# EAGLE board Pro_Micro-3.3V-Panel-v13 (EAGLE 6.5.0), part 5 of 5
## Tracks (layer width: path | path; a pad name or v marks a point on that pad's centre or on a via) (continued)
VCC  (via drill 0.25) (continued)
  Top 0.203: SJ1.2 7.72,37.75 8.13,37.34 8.76,37.34 9.21,36.89 11.37,36.89 12.06,36.2 12.06,35.52 R2.2 12.78,34.78 R11.2 11.93,32.51 C13.A | C3.2 20.51,15.84 20.85,15.49 20.85,13.22 D3.A | 11.14,13.88 C10.1 | 11.38,12.48 D1.A 11.32,12.55 C10.1 | 11.99,19.17 11.59,18.76 11.33,18.76 10.55,17.98 v10.55,16.75 10.41,16.61 10.41,14.78 C10.1 | 19.82,15.84 C3.2 | 17.06,16.73 17.39,16.4 17.39,14.94 arc90 17.44,14.88 | U3.34 20.33,21.92 21.33,21.92 v21.34,21.94 | C13.A 12.31,30.11 | 15.95,27.65 15.95,29.96 15.59,30.32 13.61,30.32 13.4,30.11 C13.A | 15.95,27.65 arc90 15.84,27.76 U2.5 | 17.14,27.19 18.2,27.19 18.41,26.98 18.41,26.5 18.69,26.22 20.82,26.22 v21.51,26.92 23.04,28.45 JP6.4 23.23,28.45 | 17.14,27.19 16.18,27.19 15.95,27.42 15.95,27.65 | 17.14,27.19 17.07,27.12 17.07,25.64 16.71,25.28 | v16.55,14.88 17.44,14.88 | 17.44,14.88 19.11,14.88 C3.2
  Bottom 0.203: v10.55,16.75 10.41,16.61 10.41,15.49 10.97,14.93 10.97,13.48 11.4,13.05 14.43,13.05 16.27,14.88 v16.55,14.88 arc90 v16.56,14.89 16.56,19.27 14.83,21 14.83,21.41 15.56,22.14 15.94,22.14 16.94,23.14 17.12,23.14 17.59,22.67 | v21.34,21.94 20.61,21.94 20.52,22.03 18.23,22.03 17.59,22.67 | v21.51,26.92 21.51,26.59 17.59,22.67
VCC1  (via drill 0.25)
  Top 0.203: SJ2.2 26,37.75 26.42,37.34 27.05,37.34 27.5,36.89 29.65,36.89 30.35,36.2 30.35,35.52 R3.2 31.06,34.78 R1.2 30.21,32.51 C8.A | C9.2 38.8,15.84 39.14,15.49 39.14,13.22 D4.A | 29.43,13.88 C7.1 | 29.67,12.48 D5.A 29.6,12.55 C7.1 | 30.28,19.17 29.88,18.76 29.62,18.76 28.84,17.98 v28.84,16.75 28.7,16.61 28.7,14.78 C7.1 | 38.11,15.84 C9.2 | 35.35,16.73 35.67,16.4 35.67,14.94 arc90 35.73,14.88 | U4.34 38.61,21.92 39.61,21.92 v39.63,21.94 | C8.A 30.6,30.11 | 34.23,27.65 34.23,29.96 33.87,30.32 31.9,30.32 31.68,30.11 C8.A | 34.23,27.65 arc90 34.12,27.76 U1.5 | 35.42,27.19 36.49,27.19 36.7,26.98 36.7,26.5 36.98,26.22 39.11,26.22 v39.8,26.92 41.33,28.45 JP3.4 41.52,28.45 | 35.42,27.19 34.47,27.19 34.23,27.42 34.23,27.65 | 35.42,27.19 35.36,27.12 35.36,25.64 35,25.28 | v34.84,14.88 35.73,14.88 | 35.73,14.88 37.4,14.88 C9.2
  Bottom 0.203: v28.84,16.75 28.7,16.61 28.7,15.49 29.26,14.93 29.26,13.48 29.69,13.05 32.72,13.05 34.55,14.88 v34.84,14.88 arc90 34.84,14.89 34.84,19.27 33.12,21 33.12,21.41 33.85,22.14 34.23,22.14 35.23,23.14 35.41,23.14 35.88,22.67 | v39.63,21.94 38.9,21.94 38.81,22.03 36.52,22.03 35.88,22.67 | v39.8,26.92 39.8,26.59 35.88,22.67
VCC2  (via drill 0.25)
  Top 0.203: SJ3.2 44.29,37.75 44.7,37.34 45.34,37.34 45.78,36.89 47.94,36.89 48.64,36.2 48.64,35.52 R14.2 49.35,34.78 R13.2 48.5,32.51 C20.A | C21.2 57.09,15.84 57.43,15.49 57.43,13.22 D7.A | 47.71,13.88 C18.1 | 47.95,12.48 D8.A 47.89,12.55 C18.1 | 48.57,19.17 48.16,18.76 47.91,18.76 47.13,17.98 v47.13,16.75 46.99,16.61 46.99,14.78 C18.1 | 56.4,15.84 C21.2 | 53.64,16.73 53.96,16.4 53.96,14.94 arc90 54.02,14.88 | U6.34 56.9,21.92 57.9,21.92 v57.92,21.94 | C20.A 48.88,30.11 | 52.52,27.65 52.52,29.96 52.16,30.32 50.19,30.32 49.97,30.11 C20.A | 52.52,27.65 arc90 52.41,27.76 U5.5 | 53.71,27.19 54.78,27.19 54.99,26.98 54.99,26.5 55.26,26.22 57.39,26.22 v58.09,26.92 59.62,28.45 JP9.4 59.81,28.45 | 53.71,27.19 52.75,27.19 52.52,27.42 52.52,27.65 | 53.71,27.19 53.65,27.12 53.65,25.64 53.29,25.28 | v53.12,14.88 54.02,14.88 | 54.02,14.88 55.69,14.88 C21.2
  Bottom 0.203: v47.13,16.75 46.99,16.61 46.99,15.49 47.55,14.93 47.55,13.48 47.98,13.05 51.01,13.05 52.84,14.88 v53.12,14.88 arc90 53.13,14.89 53.13,19.27 51.41,21 51.41,21.41 52.14,22.14 52.52,22.14 53.52,23.14 53.69,23.14 54.17,22.67 | v57.92,21.94 57.19,21.94 57.1,22.03 54.81,22.03 54.17,22.67 | v58.09,26.92 58.09,26.59 54.17,22.67
VCC3  (via drill 0.25)
  Top 0.203: SJ4.2 62.58,37.75 62.99,37.34 63.63,37.34 64.07,36.89 66.23,36.89 66.93,36.2 66.93,35.52 R20.2 67.64,34.78 R19.2 66.79,32.51 C29.A | C30.2 75.38,15.84 75.72,15.49 75.72,13.22 D10.A | 66,13.88 C28.1 | 66.24,12.48 D11.A 66.18,12.55 C28.1 | 66.86,19.17 66.45,18.76 66.2,18.76 65.42,17.98 v65.42,16.75 65.28,16.61 65.28,14.78 C28.1 | 74.69,15.84 C30.2 | 71.92,16.73 72.25,16.4 72.25,14.94 arc90 72.31,14.88 | U8.34 75.19,21.92 76.19,21.92 v76.21,21.94 | C29.A 67.17,30.11 | 70.81,27.65 70.81,29.96 70.45,30.32 68.47,30.32 68.26,30.11 C29.A | 70.81,27.65 arc90 70.7,27.76 U7.5 | 72,27.19 73.07,27.19 73.27,26.98 73.27,26.5 73.55,26.22 75.68,26.22 v76.38,26.92 77.91,28.45 JP13.4 78.09,28.45 | 72,27.19 71.04,27.19 70.81,27.42 70.81,27.65 | 72,27.19 71.94,27.12 71.94,25.64 71.58,25.28 | v71.41,14.88 72.31,14.88 | 72.31,14.88 73.97,14.88 C30.2
  Bottom 0.203: v65.42,16.75 65.28,16.61 65.28,15.49 65.84,14.93 65.84,13.48 66.27,13.05 69.3,13.05 71.13,14.88 v71.41,14.88 arc90 v71.42,14.89 71.42,19.27 69.69,21 69.69,21.41 70.43,22.14 70.81,22.14 71.8,23.14 71.98,23.14 72.45,22.67 | v76.21,21.94 75.48,21.94 75.39,22.03 73.1,22.03 72.45,22.67 | v76.38,26.92 76.38,26.59 72.45,22.67
VCC4  (via drill 0.25)
  Top 0.203: SJ5.2 80.87,37.75 81.28,37.34 81.92,37.34 82.36,36.89 84.52,36.89 85.22,36.2 85.22,35.52 R26.2 85.93,34.78 R25.2 85.08,32.51 C38.A | C39.2 93.66,15.84 94,15.49 94,13.22 D13.A | 84.29,13.88 C37.1 | 84.53,12.48 D14.A 84.47,12.55 C37.1 | 85.15,19.17 84.74,18.76 84.48,18.76 83.71,17.98 v83.71,16.75 83.57,16.61 83.57,14.78 C37.1 | 92.98,15.84 C39.2 | 90.21,16.73 90.54,16.4 90.54,14.94 arc90 90.59,14.88 | U10.34 93.48,21.92 94.48,21.92 v94.5,21.94 | C38.A 85.46,30.11 | 89.1,27.65 89.1,29.96 88.74,30.32 86.76,30.32 86.55,30.11 C38.A | 89.1,27.65 arc90 88.99,27.76 U9.5 | 90.29,27.19 91.36,27.19 91.56,26.98 91.56,26.5 91.84,26.22 93.97,26.22 v94.66,26.92 96.19,28.45 JP17.4 96.38,28.45 | 90.29,27.19 89.33,27.19 89.1,27.42 89.1,27.65 | 90.29,27.19 90.23,27.12 90.23,25.64 89.86,25.28 | v89.7,14.88 90.59,14.88 | 90.59,14.88 92.26,14.88 C39.2
  Bottom 0.203: v83.71,16.75 83.57,16.61 83.57,15.49 84.12,14.93 84.12,13.48 84.55,13.05 87.58,13.05 89.42,14.88 v89.7,14.88 arc90 v89.71,14.89 89.71,19.27 87.98,21 87.98,21.41 88.72,22.14 89.09,22.14 90.09,23.14 90.27,23.14 90.74,22.67 | v94.5,21.94 93.76,21.94 93.67,22.03 91.38,22.03 90.74,22.67 | v94.66,26.92 94.66,26.59 90.74,22.67
VCC5  (via drill 0.25)
  Top 0.203: SJ6.2 99.16,37.75 99.57,37.34 100.2,37.34 100.65,36.89 102.81,36.89 103.5,36.2 103.5,35.52 R32.2 104.22,34.78 R31.2 103.36,32.51 C47.A | C48.2 111.95,15.84 112.29,15.49 112.29,13.22 D16.A | 102.58,13.88 C46.1 | 102.82,12.48 D17.A 102.76,12.55 C46.1 | 103.43,19.17 103.03,18.76 102.77,18.76 101.99,17.98 v101.99,16.75 101.85,16.61 101.85,14.78 C46.1 | 111.26,15.84 C48.2 | 108.5,16.73 108.83,16.4 108.83,14.94 arc90 108.88,14.88 | U12.34 111.77,21.92 112.77,21.92 v112.78,21.94 | C47.A 103.75,30.11 | 107.39,27.65 107.39,29.96 107.03,30.32 105.05,30.32 104.84,30.11 C47.A | 107.39,27.65 arc90 107.28,27.76 U11.5 | 108.58,27.19 109.64,27.19 109.85,26.98 109.85,26.5 110.13,26.22 112.26,26.22 v112.95,26.92 114.48,28.45 JP21.4 114.67,28.45 | 108.58,27.19 107.62,27.19 107.39,27.42 107.39,27.65 | 108.58,27.19 108.51,27.12 108.51,25.64 108.15,25.28 | v107.99,14.88 108.88,14.88 | 108.88,14.88 110.55,14.88 C48.2
  Bottom 0.203: v101.99,16.75 101.85,16.61 101.85,15.49 102.41,14.93 102.41,13.48 102.84,13.05 105.87,13.05 107.7,14.88 v107.99,14.88 arc90 v108,14.89 108,19.27 106.27,21 106.27,21.41 107,22.14 107.38,22.14 108.38,23.14 108.56,23.14 109.03,22.67 | v112.78,21.94 112.05,21.94 111.96,22.03 109.67,22.03 109.03,22.67 | v112.95,26.92 112.95,26.59 109.03,22.67
VCC6  (via drill 0.25)
  Top 0.203: SJ7.2 7.72,74.58 8.13,74.17 8.76,74.17 9.21,73.72 11.37,73.72 12.06,73.03 12.06,72.35 R38.2 12.78,71.61 R37.2 11.93,69.34 C56.A | C57.2 20.51,52.67 20.85,52.32 20.85,50.05 D19.A | 11.14,50.71 C55.1 | 11.38,49.31 D20.A 11.32,49.38 C55.1 | 11.99,56 11.59,55.59 11.33,55.59 10.55,54.81 v10.55,53.58 10.41,53.44 10.41,51.61 C55.1 | 19.82,52.67 C57.2 | 17.06,53.56 17.39,53.23 17.39,51.77 arc90 17.44,51.71 | U14.34 20.33,58.75 21.33,58.75 v21.34,58.77 | C56.A 12.31,66.94 | 15.95,64.48 15.95,66.79 15.59,67.15 13.61,67.15 13.4,66.94 C56.A | 15.95,64.48 arc90 15.84,64.59 U13.5 | 17.14,64.02 18.2,64.02 18.41,63.81 18.41,63.33 18.69,63.05 20.82,63.05 v21.51,63.75 23.04,65.28 JP25.4 23.23,65.28 | 17.14,64.02 16.18,64.02 15.95,64.25 15.95,64.48 | 17.14,64.02 17.07,63.95 17.07,62.47 16.71,62.11 | v16.55,51.71 17.44,51.71 | 17.44,51.71 19.11,51.71 C57.2
  Bottom 0.203: v10.55,53.58 10.41,53.44 10.41,52.32 10.97,51.76 10.97,50.31 11.4,49.88 14.43,49.88 16.27,51.71 v16.55,51.71 arc90 v16.56,51.72 16.56,56.1 14.83,57.83 14.83,58.24 15.56,58.97 15.94,58.97 16.94,59.97 17.12,59.97 17.59,59.5 | v21.34,58.77 20.61,58.77 20.52,58.86 18.23,58.86 17.59,59.5 | v21.51,63.75 21.51,63.42 17.59,59.5
VCC7  (via drill 0.25)
  Top 0.203: SJ8.2 26,74.58 26.42,74.17 27.05,74.17 27.5,73.72 29.65,73.72 30.35,73.03 30.35,72.35 R44.2 31.06,71.61 R43.2 30.21,69.34 C65.A | C66.2 38.8,52.67 39.14,52.32 39.14,50.05 D22.A | 29.43,50.71 C64.1 | 29.67,49.31 D23.A 29.6,49.38 C64.1 | 30.28,56 29.88,55.59 29.62,55.59 28.84,54.81 v28.84,53.58 28.7,53.44 28.7,51.61 C64.1 | 38.11,52.67 C66.2 | 35.35,53.56 35.67,53.23 35.67,51.77 arc90 35.73,51.71 | U16.34 38.61,58.75 39.61,58.75 v39.63,58.77 | C65.A 30.6,66.94 | 34.23,64.48 34.23,66.79 33.87,67.15 31.9,67.15 31.68,66.94 C65.A | 34.23,64.48 arc90 34.12,64.59 U15.5 | 35.42,64.02 36.49,64.02 36.7,63.81 36.7,63.33 36.98,63.05 39.11,63.05 v39.8,63.75 41.33,65.28 JP29.4 41.52,65.28 | 35.42,64.02 34.47,64.02 34.23,64.25 34.23,64.48 | 35.42,64.02 35.36,63.95 35.36,62.47 35,62.11 | v34.84,51.71 35.73,51.71 | 35.73,51.71 37.4,51.71 C66.2
  Bottom 0.203: v28.84,53.58 28.7,53.44 28.7,52.32 29.26,51.76 29.26,50.31 29.69,49.88 32.72,49.88 34.55,51.71 v34.84,51.71 arc90 34.84,51.72 34.84,56.1 33.12,57.83 33.12,58.24 33.85,58.97 34.23,58.97 35.23,59.97 35.41,59.97 35.88,59.5 | v39.63,58.77 38.9,58.77 38.81,58.86 36.52,58.86 35.88,59.5 | v39.8,63.75 39.8,63.42 35.88,59.5
VCC8  (via drill 0.25)
  Top 0.203: SJ9.2 44.29,74.58 44.7,74.17 45.34,74.17 45.78,73.72 47.94,73.72 48.64,73.03 48.64,72.35 R50.2 49.35,71.61 R49.2 48.5,69.34 C74.A | C75.2 57.09,52.67 57.43,52.32 57.43,50.05 D25.A | 47.71,50.71 C73.1 | 47.95,49.31 D26.A 47.89,49.38 C73.1 | 48.57,56 48.16,55.59 47.91,55.59 47.13,54.81 v47.13,53.58 46.99,53.44 46.99,51.61 C73.1 | 56.4,52.67 C75.2 | 53.64,53.56 53.96,53.23 53.96,51.77 arc90 54.02,51.71 | U18.34 56.9,58.75 57.9,58.75 v57.92,58.77 | C74.A 48.88,66.94 | 52.52,64.48 52.52,66.79 52.16,67.15 50.19,67.15 49.97,66.94 C74.A | 52.52,64.48 arc90 52.41,64.59 U17.5 | 53.71,64.02 54.78,64.02 54.99,63.81 54.99,63.33 55.26,63.05 57.39,63.05 v58.09,63.75 59.62,65.28 JP33.4 59.81,65.28 | 53.71,64.02 52.75,64.02 52.52,64.25 52.52,64.48 | 53.71,64.02 53.65,63.95 53.65,62.47 53.29,62.11 | v53.12,51.71 54.02,51.71 | 54.02,51.71 55.69,51.71 C75.2
  Bottom 0.203: v47.13,53.58 46.99,53.44 46.99,52.32 47.55,51.76 47.55,50.31 47.98,49.88 51.01,49.88 52.84,51.71 v53.12,51.71 arc90 53.13,51.72 53.13,56.1 51.41,57.83 51.41,58.24 52.14,58.97 52.52,58.97 53.52,59.97 53.69,59.97 54.17,59.5 | v57.92,58.77 57.19,58.77 57.1,58.86 54.81,58.86 54.17,59.5 | v58.09,63.75 58.09,63.42 54.17,59.5
VCC9  (via drill 0.25)
  Top 0.203: SJ10.2 62.58,74.58 62.99,74.17 63.63,74.17 64.07,73.72 66.23,73.72 66.93,73.03 66.93,72.35 R56.2 67.64,71.61 R55.2 66.79,69.34 C83.A | C84.2 75.38,52.67 75.72,52.32 75.72,50.05 D28.A | 66,50.71 C82.1 | 66.24,49.31 D29.A 66.18,49.38 C82.1 | 66.86,56 66.45,55.59 66.2,55.59 65.42,54.81 v65.42,53.58 65.28,53.44 65.28,51.61 C82.1 | 74.69,52.67 C84.2 | 71.92,53.56 72.25,53.23 72.25,51.77 arc90 72.31,51.71 | U20.34 75.19,58.75 76.19,58.75 v76.21,58.77 | C83.A 67.17,66.94 | 70.81,64.48 70.81,66.79 70.45,67.15 68.47,67.15 68.26,66.94 C83.A | 70.81,64.48 arc90 70.7,64.59 U19.5 | 72,64.02 73.07,64.02 73.27,63.81 73.27,63.33 73.55,63.05 75.68,63.05 v76.38,63.75 77.91,65.28 JP37.4 78.09,65.28 | 72,64.02 71.04,64.02 70.81,64.25 70.81,64.48 | 72,64.02 71.94,63.95 71.94,62.47 71.58,62.11 | v71.41,51.71 72.31,51.71 | 72.31,51.71 73.97,51.71 C84.2
  Bottom 0.203: v65.42,53.58 65.28,53.44 65.28,52.32 65.84,51.76 65.84,50.31 66.27,49.88 69.3,49.88 71.13,51.71 v71.41,51.71 arc90 v71.42,51.72 71.42,56.1 69.69,57.83 69.69,58.24 70.43,58.97 70.81,58.97 71.8,59.97 71.98,59.97 72.45,59.5 | v76.21,58.77 75.48,58.77 75.39,58.86 73.1,58.86 72.45,59.5 | v76.38,63.75 76.38,63.42 72.45,59.5
VCC10  (via drill 0.25)
  Top 0.203: SJ11.2 80.87,74.58 81.28,74.17 81.92,74.17 82.36,73.72 84.52,73.72 85.22,73.03 85.22,72.35 R62.2 85.93,71.61 R61.2 85.08,69.34 C92.A | C93.2 93.66,52.67 94,52.32 94,50.05 D31.A | 84.29,50.71 C91.1 | 84.53,49.31 D32.A 84.47,49.38 C91.1 | 85.15,56 84.74,55.59 84.48,55.59 83.71,54.81 v83.71,53.58 83.57,53.44 83.57,51.61 C91.1 | 92.98,52.67 C93.2 | 90.21,53.56 90.54,53.23 90.54,51.77 arc90 90.59,51.71 | U22.34 93.48,58.75 94.48,58.75 v94.5,58.77 | C92.A 85.46,66.94 | 89.1,64.48 89.1,66.79 88.74,67.15 86.76,67.15 86.55,66.94 C92.A | 89.1,64.48 arc90 88.99,64.59 U21.5 | 90.29,64.02 91.36,64.02 91.56,63.81 91.56,63.33 91.84,63.05 93.97,63.05 v94.66,63.75 96.19,65.28 JP41.4 96.38,65.28 | 90.29,64.02 89.33,64.02 89.1,64.25 89.1,64.48 | 90.29,64.02 90.23,63.95 90.23,62.47 89.86,62.11 | v89.7,51.71 90.59,51.71 | 90.59,51.71 92.26,51.71 C93.2
  Bottom 0.203: v83.71,53.58 83.57,53.44 83.57,52.32 84.12,51.76 84.12,50.31 84.55,49.88 87.58,49.88 89.42,51.71 v89.7,51.71 arc90 v89.71,51.72 89.71,56.1 87.98,57.83 87.98,58.24 88.72,58.97 89.09,58.97 90.09,59.97 90.27,59.97 90.74,59.5 | v94.5,58.77 93.76,58.77 93.67,58.86 91.38,58.86 90.74,59.5 | v94.66,63.75 94.66,63.42 90.74,59.5
VCC11  (via drill 0.25)
  Top 0.203: SJ12.2 99.16,74.58 99.57,74.17 100.2,74.17 100.65,73.72 102.81,73.72 103.5,73.03 103.5,72.35 R68.2 104.22,71.61 R67.2 103.36,69.34 C101.A | C102.2 111.95,52.67 112.29,52.32 112.29,50.05 D34.A | 102.58,50.71 C100.1 | 102.82,49.31 D35.A 102.76,49.38 C100.1 | 103.43,56 103.03,55.59 102.77,55.59 101.99,54.81 v101.99,53.58 101.85,53.44 101.85,51.61 C100.1 | 111.26,52.67 C102.2 | 108.5,53.56 108.83,53.23 108.83,51.77 arc90 108.88,51.71 | U24.34 111.77,58.75 112.77,58.75 v112.78,58.77 | C101.A 103.75,66.94 | 107.39,64.48 107.39,66.79 107.03,67.15 105.05,67.15 104.84,66.94 C101.A | 107.39,64.48 arc90 107.28,64.59 U23.5 | 108.58,64.02 109.64,64.02 109.85,63.81 109.85,63.33 110.13,63.05 112.26,63.05 v112.95,63.75 114.48,65.28 JP45.4 114.67,65.28 | 108.58,64.02 107.62,64.02 107.39,64.25 107.39,64.48 | 108.58,64.02 108.51,63.95 108.51,62.47 108.15,62.11 | v107.99,51.71 108.88,51.71 | 108.88,51.71 110.55,51.71 C102.2
  Bottom 0.203: v101.99,53.58 101.85,53.44 101.85,52.32 102.41,51.76 102.41,50.31 102.84,49.88 105.87,49.88 107.7,51.71 v107.99,51.71 arc90 v108,51.72 108,56.1 106.27,57.83 106.27,58.24 107,58.97 107.38,58.97 108.38,59.97 108.56,59.97 109.03,59.5 | v112.78,58.77 112.05,58.77 111.96,58.86 109.67,58.86 109.03,59.5 | v112.95,63.75 112.95,63.42 109.03,59.5
VCC12  (via drill 0.25)
  Top 0.203: SJ13.2 7.72,111.41 8.13,111 8.76,111 9.21,110.55 11.37,110.55 12.06,109.86 12.06,109.18 R74.2 12.78,108.44 R73.2 11.93,106.17 C110.A | C111.2 20.51,89.5 20.85,89.15 20.85,86.88 D37.A | 11.14,87.54 C109.1 | 11.38,86.14 D38.A 11.32,86.21 C109.1 | 11.99,92.83 11.59,92.42 11.33,92.42 10.55,91.64 v10.55,90.41 10.41,90.27 10.41,88.44 C109.1 | 19.82,89.5 C111.2 | 17.06,90.39 17.39,90.06 17.39,88.6 arc90 17.44,88.54 | U26.34 20.33,95.58 21.33,95.58 v21.34,95.6 | C110.A 12.31,103.77 | 15.95,101.31 15.95,103.62 15.59,103.98 13.61,103.98 13.4,103.77 C110.A | 15.95,101.31 arc90 15.84,101.42 U25.5 | 17.14,100.85 18.2,100.85 18.41,100.64 18.41,100.16 18.69,99.88 20.82,99.88 v21.51,100.58 23.04,102.11 JP49.4 23.23,102.11 | 17.14,100.85 16.18,100.85 15.95,101.08 15.95,101.31 | 17.14,100.85 17.07,100.78 17.07,99.3 16.71,98.94 | v16.55,88.54 17.44,88.54 | 17.44,88.54 19.11,88.54 C111.2
  Bottom 0.203: v10.55,90.41 10.41,90.27 10.41,89.15 10.97,88.59 10.97,87.14 11.4,86.71 14.43,86.71 16.27,88.54 v16.55,88.54 arc90 v16.56,88.55 16.56,92.93 14.83,94.66 14.83,95.07 15.56,95.8 15.94,95.8 16.94,96.8 17.12,96.8 17.59,96.33 | v21.34,95.6 20.61,95.6 20.52,95.69 18.23,95.69 17.59,96.33 | v21.51,100.58 21.51,100.25 17.59,96.33
VCC13  (via drill 0.25)
  Top 0.203: SJ14.2 26,111.41 26.42,111 27.05,111 27.5,110.55 29.65,110.55 30.35,109.86 30.35,109.18 R80.2 31.06,108.44 R79.2 30.21,106.17 C119.A | C120.2 38.8,89.5 39.14,89.15 39.14,86.88 D40.A | 29.43,87.54 C118.1 | 29.67,86.14 D41.A 29.6,86.21 C118.1 | 30.28,92.83 29.88,92.42 29.62,92.42 28.84,91.64 v28.84,90.41 28.7,90.27 28.7,88.44 C118.1 | 38.11,89.5 C120.2 | 35.35,90.39 35.67,90.06 35.67,88.6 arc90 35.73,88.54 | U28.34 38.61,95.58 39.61,95.58 v39.63,95.6 | C119.A 30.6,103.77 | 34.23,101.31 34.23,103.62 33.87,103.98 31.9,103.98 31.68,103.77 C119.A | 34.23,101.31 arc90 34.12,101.42 U27.5 | 35.42,100.85 36.49,100.85 36.7,100.64 36.7,100.16 36.98,99.88 39.11,99.88 v39.8,100.58 41.33,102.11 JP53.4 41.52,102.11 | 35.42,100.85 34.47,100.85 34.23,101.08 34.23,101.31 | 35.42,100.85 35.36,100.78 35.36,99.3 35,98.94 | v34.84,88.54 35.73,88.54 | 35.73,88.54 37.4,88.54 C120.2
  Bottom 0.203: v28.84,90.41 28.7,90.27 28.7,89.15 29.26,88.59 29.26,87.14 29.69,86.71 32.72,86.71 34.55,88.54 v34.84,88.54 arc90 34.84,88.55 34.84,92.93 33.12,94.66 33.12,95.07 33.85,95.8 34.23,95.8 35.23,96.8 35.41,96.8 35.88,96.33 | v39.63,95.6 38.9,95.6 38.81,95.69 36.52,95.69 35.88,96.33 | v39.8,100.58 39.8,100.25 35.88,96.33
VCC14  (via drill 0.25)
  Top 0.203: SJ15.2 44.29,111.41 44.7,111 45.34,111 45.78,110.55 47.94,110.55 48.64,109.86 48.64,109.18 R86.2 49.35,108.44 R85.2 48.5,106.17 C128.A | C129.2 57.09,89.5 57.43,89.15 57.43,86.88 D43.A | 47.71,87.54 C127.1 | 47.95,86.14 D44.A 47.89,86.21 C127.1 | 48.57,92.83 48.16,92.42 47.91,92.42 47.13,91.64 v47.13,90.41 46.99,90.27 46.99,88.44 C127.1 | 56.4,89.5 C129.2 | 53.64,90.39 53.96,90.06 53.96,88.6 arc90 54.02,88.54 | U30.34 56.9,95.58 57.9,95.58 v57.92,95.6 | C128.A 48.88,103.77 | 52.52,101.31 52.52,103.62 52.16,103.98 50.19,103.98 49.97,103.77 C128.A | 52.52,101.31 arc90 52.41,101.42 U29.5 | 53.71,100.85 54.78,100.85 54.99,100.64 54.99,100.16 55.26,99.88 57.39,99.88 v58.09,100.58 59.62,102.11 JP57.4 59.81,102.11 | 53.71,100.85 52.75,100.85 52.52,101.08 52.52,101.31 | 53.71,100.85 53.65,100.78 53.65,99.3 53.29,98.94 | v53.12,88.54 54.02,88.54 | 54.02,88.54 55.69,88.54 C129.2
  Bottom 0.203: v47.13,90.41 46.99,90.27 46.99,89.15 47.55,88.59 47.55,87.14 47.98,86.71 51.01,86.71 52.84,88.54 v53.12,88.54 arc90 53.13,88.55 53.13,92.93 51.41,94.66 51.41,95.07 52.14,95.8 52.52,95.8 53.52,96.8 53.69,96.8 54.17,96.33 | v57.92,95.6 57.19,95.6 57.1,95.69 54.81,95.69 54.17,96.33 | v58.09,100.58 58.09,100.25 54.17,96.33
VCC15  (via drill 0.25)
  Top 0.203: SJ16.2 62.58,111.41 62.99,111 63.63,111 64.07,110.55 66.23,110.55 66.93,109.86 66.93,109.18 R92.2 67.64,108.44 R91.2 66.79,106.17 C137.A | C138.2 75.38,89.5 75.72,89.15 75.72,86.88 D46.A | 66,87.54 C136.1 | 66.24,86.14 D47.A 66.18,86.21 C136.1 | 66.86,92.83 66.45,92.42 66.2,92.42 65.42,91.64 v65.42,90.41 65.28,90.27 65.28,88.44 C136.1 | 74.69,89.5 C138.2 | 71.92,90.39 72.25,90.06 72.25,88.6 arc90 72.31,88.54 | U32.34 75.19,95.58 76.19,95.58 v76.21,95.6 | C137.A 67.17,103.77 | 70.81,101.31 70.81,103.62 70.45,103.98 68.47,103.98 68.26,103.77 C137.A | 70.81,101.31 arc90 70.7,101.42 U31.5 | 72,100.85 73.07,100.85 73.27,100.64 73.27,100.16 73.55,99.88 75.68,99.88 v76.38,100.58 77.91,102.11 JP61.4 78.09,102.11 | 72,100.85 71.04,100.85 70.81,101.08 70.81,101.31 | 72,100.85 71.94,100.78 71.94,99.3 71.58,98.94 | v71.41,88.54 72.31,88.54 | 72.31,88.54 73.97,88.54 C138.2
  Bottom 0.203: v65.42,90.41 65.28,90.27 65.28,89.15 65.84,88.59 65.84,87.14 66.27,86.71 69.3,86.71 71.13,88.54 v71.41,88.54 arc90 v71.42,88.55 71.42,92.93 69.69,94.66 69.69,95.07 70.43,95.8 70.81,95.8 71.8,96.8 71.98,96.8 72.45,96.33 | v76.21,95.6 75.48,95.6 75.39,95.69 73.1,95.69 72.45,96.33 | v76.38,100.58 76.38,100.25 72.45,96.33
VCC16  (via drill 0.25)
  Top 0.203: SJ17.2 80.87,111.41 81.28,111 81.92,111 82.36,110.55 84.52,110.55 85.22,109.86 85.22,109.18 R98.2 85.93,108.44 R97.2 85.08,106.17 C146.A | C147.2 93.66,89.5 94,89.15 94,86.88 D49.A | 84.29,87.54 C145.1 | 84.53,86.14 D50.A 84.47,86.21 C145.1 | 85.15,92.83 84.74,92.42 84.48,92.42 83.71,91.64 v83.71,90.41 83.57,90.27 83.57,88.44 C145.1 | 92.98,89.5 C147.2 | 90.21,90.39 90.54,90.06 90.54,88.6 arc90 90.59,88.54 | U34.34 93.48,95.58 94.48,95.58 v94.5,95.6 | C146.A 85.46,103.77 | 89.1,101.31 89.1,103.62 88.74,103.98 86.76,103.98 86.55,103.77 C146.A | 89.1,101.31 arc90 88.99,101.42 U33.5 | 90.29,100.85 91.36,100.85 91.56,100.64 91.56,100.16 91.84,99.88 93.97,99.88 v94.66,100.58 96.19,102.11 JP65.4 96.38,102.11 | 90.29,100.85 89.33,100.85 89.1,101.08 89.1,101.31 | 90.29,100.85 90.23,100.78 90.23,99.3 89.86,98.94 | v89.7,88.54 90.59,88.54 | 90.59,88.54 92.26,88.54 C147.2
  Bottom 0.203: v83.71,90.41 83.57,90.27 83.57,89.15 84.12,88.59 84.12,87.14 84.55,86.71 87.58,86.71 89.42,88.54 v89.7,88.54 arc90 v89.71,88.55 89.71,92.93 87.98,94.66 87.98,95.07 88.72,95.8 89.09,95.8 90.09,96.8 90.27,96.8 90.74,96.33 | v94.5,95.6 93.76,95.6 93.67,95.69 91.38,95.69 90.74,96.33 | v94.66,100.58 94.66,100.25 90.74,96.33
VCC17  (via drill 0.25)
  Top 0.203: SJ18.2 99.16,111.41 99.57,111 100.2,111 100.65,110.55 102.81,110.55 103.5,109.86 103.5,109.18 R104.2 104.22,108.44 R103.2 103.36,106.17 C155.A | C156.2 111.95,89.5 112.29,89.15 112.29,86.88 D52.A | 102.58,87.54 C154.1 | 102.82,86.14 D53.A 102.76,86.21 C154.1 | 103.43,92.83 103.03,92.42 102.77,92.42 101.99,91.64 v101.99,90.41 101.85,90.27 101.85,88.44 C154.1 | 111.26,89.5 C156.2 | 108.5,90.39 108.83,90.06 108.83,88.6 arc90 108.88,88.54 | U36.34 111.77,95.58 112.77,95.58 v112.78,95.6 | C155.A 103.75,103.77 | 107.39,101.31 107.39,103.62 107.03,103.98 105.05,103.98 104.84,103.77 C155.A | 107.39,101.31 arc90 107.28,101.42 U35.5 | 108.58,100.85 109.64,100.85 109.85,100.64 109.85,100.16 110.13,99.88 112.26,99.88 v112.95,100.58 114.48,102.11 JP69.4 114.67,102.11 | 108.58,100.85 107.62,100.85 107.39,101.08 107.39,101.31 | 108.58,100.85 108.51,100.78 108.51,99.3 108.15,98.94 | v107.99,88.54 108.88,88.54 | 108.88,88.54 110.55,88.54 C156.2
  Bottom 0.203: v101.99,90.41 101.85,90.27 101.85,89.15 102.41,88.59 102.41,87.14 102.84,86.71 105.87,86.71 107.7,88.54 v107.99,88.54 arc90 v108,88.55 108,92.93 106.27,94.66 106.27,95.07 107,95.8 107.38,95.8 108.38,96.8 108.56,96.8 109.03,96.33 | v112.78,95.6 112.05,95.6 111.96,95.69 109.67,95.69 109.03,96.33 | v112.95,100.58 112.95,100.25 109.03,96.33

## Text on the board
Bottom: v13 | v13 | v13 | v13 | v13 | v13 | v13 | v13 | v13 | v13 | v13 | v13 | v13 | v13 | v13 | v13 | v13 | v13
Dimension: Route Out | Route Out | Route Out | Route Out | Route Out | Route Out | Route Out | Route Out | Route Out | Route Out
tPlace: J1 | J1 | J1 | J1 | J1 | J1 | TXO | RAW | TXO | RAW | TXO | RAW | TXO | RAW | TXO | RAW | TXO | RAW | RXI | GND | RXI | GND | RXI | GND | RXI | GND | RXI | GND | RXI | GND | GND | RST | GND | RST | GND | RST | GND | RST | GND | RST | GND | RST | GND | VCC | GND | VCC | GND | VCC | GND | VCC | GND | VCC | GND | VCC | 2 | A3 | 2 | A3 | 2 | A3 | 2 | A3 | 2 | A3 | 2 | A3 | 3 | 3 | 3 | 3 | 3 | 3 | A2 | A2 | A2 | A2 | A2 | A2 | 4 | A1 | 4 | A1 | 4 | A1 | 4 | A1 | 4 | A1 | 4 | A1 | 5 | 5 | 5 | 5 | 5 | 5 | A0 | A0 | A0 | A0 | A0 | A0 | 6 | 15 | 6 | 15 | 6 | 15 | 6 | 15 | 6 | 15 | 6 | 15 | Pro | Micro | Pro | Micro | Pro | Micro | Pro | Micro | Pro | Micro | Pro | Micro | 7 | 14 | 7 | 14 | 7 | 14 | 7 | 14 | 7 | 14 | 7 | 14 | 8 | 16 | 8 | 16 | 8 | 16 | 8 | 16 | 8 | 16 | 8 | 16 | 9 | 10 | 9 | 10 | 9 | 10 | 9 | 10 | 9 | 10 | 9 | 10 | J1 | J1 | J1 | J1 | J1 | J1 | TXO | RAW | TXO | RAW | TXO | RAW | TXO | RAW | TXO | RAW | TXO | RAW | RXI | GND | RXI | GND | RXI | GND | RXI | GND | RXI | GND | RXI | GND | GND | RST | GND | RST | GND | RST | GND | RST | GND | RST | GND | RST | GND | VCC | GND | VCC | GND | VCC | GND | VCC | GND | VCC | GND | VCC | 2 | A3 | 2 | A3 | 2 | A3 | 2 | A3 | 2 | A3 | 2 | A3 | 3 | 3 | 3 | 3 | 3 | 3 | A2 | A2 | A2 | A2 | A2 | A2 | 4 | A1 | 4 | A1 | 4 | A1 | 4 | A1 | 4 | A1 | 4 | A1 | 5 | 5 | 5 | 5 | 5 | 5 | A0 | A0 | A0 | A0 | A0 | A0 | 6 | 15 | 6 | 15 | 6 | 15 | 6 | 15 | 6 | 15 | 6 | 15 | 7 | Pro | Micro | 7 | Pro | Micro | 7 | Pro | Micro | 7 | Pro | Micro | 7 | Pro | Micro | 7 | Pro | Micro | 14 | 14 | 14 | 14 | 14 | 14 | 8 | 16 | 8 | 16 | 8 | 16 | 8 | 16 | 8 | 16 | 8 | 16 | 9 | 9 | 9 | 9 | 9 | 9 | 10 | 10 | 10 | 10 | 10 | 10 | J1 | J1 | J1 | J1 | J1 | J1 | TXO | RAW | TXO | RAW | TXO | RAW | TXO | RAW | TXO | RAW | TXO | RAW | RXI | GND | RXI | GND | RXI | GND | RXI | GND | RXI | GND | RXI | GND | GND | RST | GND | RST | GND | RST | GND | RST | GND | RST | GND | RST | GND | VCC | GND | VCC | GND | VCC | GND | VCC | GND | VCC | GND | VCC | 2 | 2 | 2 | 2 | 2 | 2 | A3 | A3 | A3 | A3 | A3 | A3 | 3 | A2 | 3 | A2 | 3 | A2 | 3 | A2 | 3 | A2 | 3 | A2 | 4 | A1 | 4 | A1 | 4 | A1 | 4 | A1 | 4 | A1 | 4 | A1 | 5 | A0 | 5 | A0 | 5 | A0 | 5 | A0 | 5 | A0 | 5 | A0 | 6 | 15 | 6 | 15 | 6 | 15 | 6 | 15 | 6 | 15 | 6 | 15 | 7 | Pro | Micro | 7 | Pro | Micro | 7 | Pro | Micro | 7 | Pro | Micro | 7 | Pro | Micro | 7 | Pro | Micro | 14 | 14 | 14 | 14 | 14 | 14 | 8 | 16 | 8 | 16 | 8 | 16 | 8 | 16 | 8 | 16 | 8 | 16 | 9 | 9 | 9 | 9 | 9 | 9 | 10 | 10 | 10 | 10 | 10 | 10
bPlace: 3.3V | 5V | 3.3V | 5V | 3.3V | 5V | 3.3V | 5V | 3.3V | 5V | 3.3V | 5V | 3.3V | 5V | 3.3V | 5V | 3.3V | 5V | 3.3V | 5V | 3.3V | 5V | 3.3V | 5V | 3.3V | 5V | 3.3V | 5V | 3.3V | 5V | 3.3V | 5V | 3.3V | 5V | 3.3V | 5V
